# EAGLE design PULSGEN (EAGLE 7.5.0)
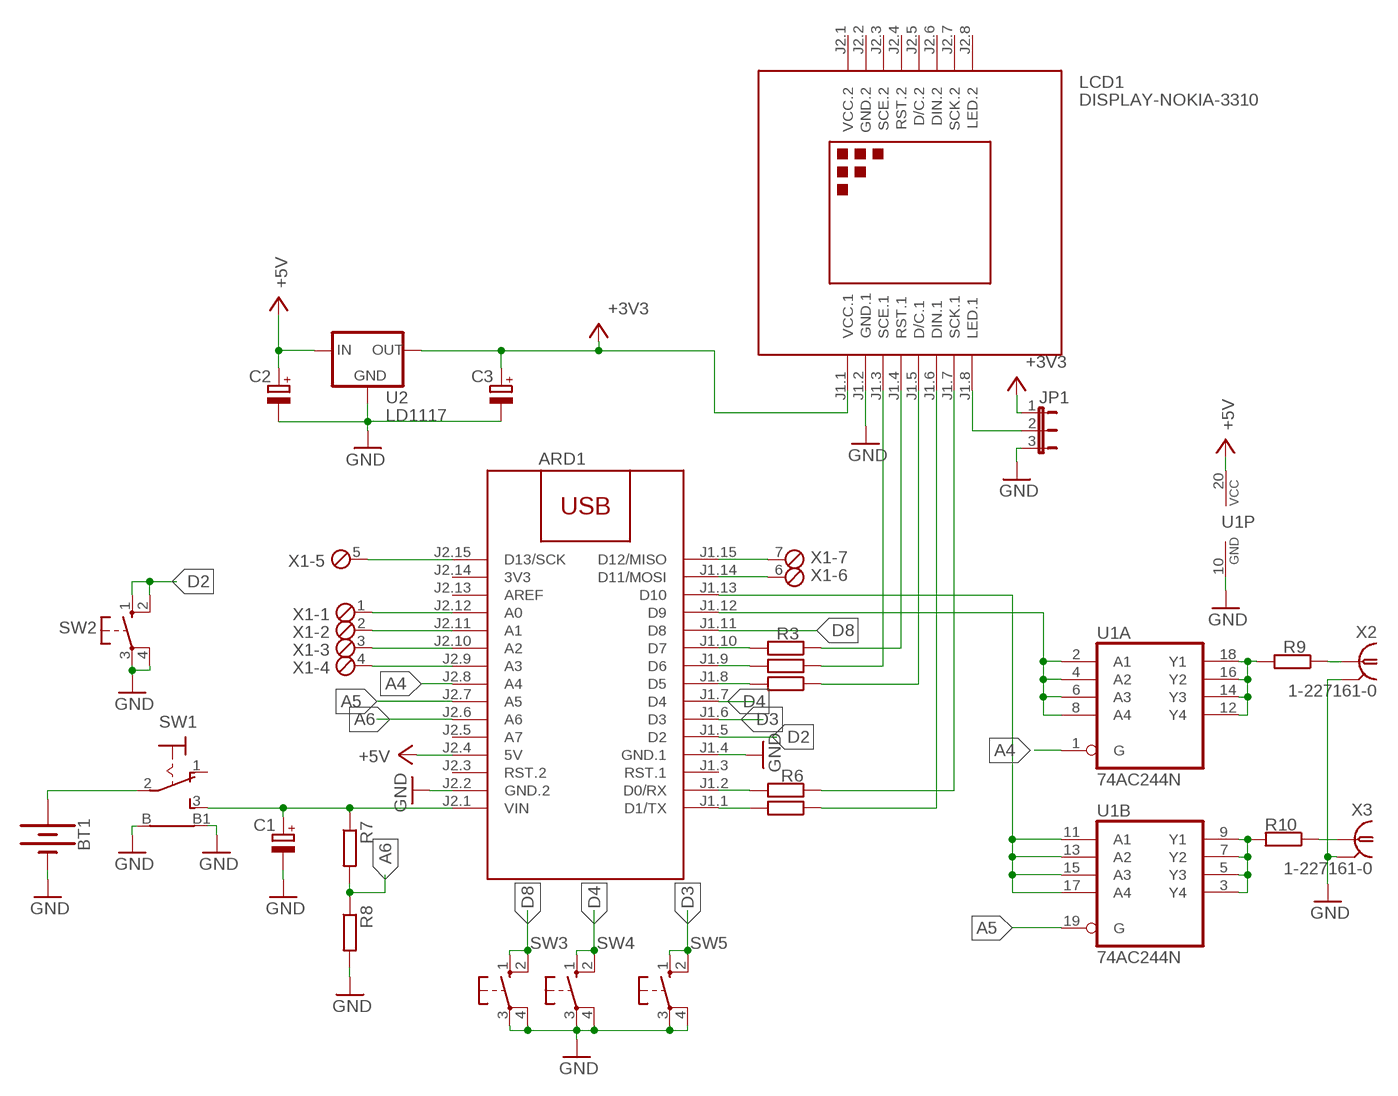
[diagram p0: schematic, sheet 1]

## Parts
ARD1  ARDUINO-NANO-3.0  [ARDUINO-NANO-3.0]
BT1  BATTERY-9V  [BATTCON_9V]
C1  CPOL-EUSMCC  [SMC_C]
C2  CPOL-EUSMCB  [SMC_B]
C3  CPOL-EUSMCB  [SMC_B]
JP1  JP2E  [JP2]
LCD1  DISPLAY-NOKIA-3310  [DISPLAY-NOKIA-3310]
R2  R-EU_R1206  [R1206]
R3  R-EU_R1206  [R1206]
R4  R-EU_R1206  [R1206]
R5  R-EU_R1206  [R1206]
R6  R-EU_R1206  [R1206]
R7  R-EU_R1206  [R1206]
R8  R-EU_R1206  [R1206]
R9  R-EU_R1206  [R1206]
R10  R-EU_R1206  [R1206]
SW1  9070-1W  [9070-1W]
SW2  40-XX  [B3F-40XX]
SW3  40-XX  [B3F-40XX]
SW4  40-XX  [B3F-40XX]
SW5  40-XX  [B3F-40XX]
U1  74AC244N  [DIL20]
U2  LD1117  [SOT223]
X1  MPT7  [7POL254]
X2  1-227161-0  [AMP_227161]
X3  1-227161-0  [AMP_227161]

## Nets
+3V3: C3.+ JP1.1 LCD1.J1.1(VCC.1) U2.2(OUT)
+5V: ARD1.J2.4(5V) C2.+ U1.20(P:VCC) U2.3(IN)
A4: ARD1.J2.8(A4) U1.1(A:G)
A5: ARD1.J2.7(A5) U1.19(B:G)
A6: ARD1.J2.6(A6) R7.2 R8.1
D2: ARD1.J1.5(D2) SW2.1(S) SW2.2(S1)
D3: ARD1.J1.6(D3) SW5.1(S) SW5.2(S1)
D4: ARD1.J1.7(D4) SW4.1(S) SW4.2(S1)
D8: ARD1.J1.11(D8) SW3.1(S) SW3.2(S1)
GND: ARD1.J1.4(GND.1) ARD1.J2.2(GND.2) BT1.- C1.- C2.- C3.- JP1.3 LCD1.J1.2(GND.1) R8.2 SW1.B SW1.B1 SW2.3(P) SW2.4(P1) SW3.3(P) SW3.4(P1) SW4.3(P) SW4.4(P1) SW5.3(P) SW5.4(P1) U1.10(P:GND) U2.1(GND) X2.2 X3.2
N$1: ARD1.J1.1(D1/TX) R5.2
N$2: LCD1.J1.6(DIN.1) R5.1
N$3: ARD1.J1.10(D7) R3.2
N$4: ARD1.J1.9(D6) R2.2
N$5: ARD1.J1.8(D5) R4.2
N$6: ARD1.J1.2(D0/RX) R6.2
N$7: ARD1.J2.12(A0) X1.1
N$8: LCD1.J1.4(RST.1) R3.1
N$9: LCD1.J1.3(SCE.1) R2.1
N$10: LCD1.J1.5(D/C.1) R4.1
N$11: ARD1.J2.11(A1) X1.2
N$12: LCD1.J1.7(SCK.1) R6.1
N$13: JP1.2 LCD1.J1.8(LED.1)
N$14: ARD1.J2.10(A2) X1.3
N$15: ARD1.J2.9(A3) X1.4
N$16: ARD1.J2.15(D13/SCK) X1.5
N$17: ARD1.J1.14(D11/MOSI) X1.6
N$18: ARD1.J1.15(D12/MISO) X1.7
N$19: R9.1 X2.1
N$20: ARD1.J1.12(D9) U1.2(A:A1) U1.4(A:A2) U1.6(A:A3) U1.8(A:A4)
N$21: ARD1.J1.13(D10) U1.11(B:A1) U1.13(B:A2) U1.15(B:A3) U1.17(B:A4)
N$22: R9.2 U1.12(A:Y4) U1.14(A:Y3) U1.16(A:Y2) U1.18(A:Y1)
N$23: R10.2 U1.3(B:Y4) U1.5(B:Y3) U1.7(B:Y2) U1.9(B:Y1)
N$24: BT1.+ SW1.2(P)
N$25: ARD1.J2.1(VIN) C1.+ R7.1 SW1.3(S)
N$26: R10.1 X3.1
Unconnected: ARD1.J1.3(RST.1) ARD1.J2.3(RST.2) ARD1.J2.5(A7) ARD1.J2.13(AREF) LCD1.J2.3(SCE.2) LCD1.J2.4(RST.2) LCD1.J2.5(D/C.2) LCD1.J2.6(DIN.2) LCD1.J2.7(SCK.2) LCD1.J2.8(LED.2) SW1.1(O)

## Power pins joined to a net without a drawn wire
3V3: ARD1.J2.14(3V3)
GND.2: LCD1.J2.2(GND.2)
VCC.2: LCD1.J2.1(VCC.2)

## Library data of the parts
ARD1 = diy-modules:ARDUINO-NANO-3.0: Arduino Nano 3.0 and compatible devices More details available here: https://www.arduino.cc/en/Main/ArduinoBoardNano Click here to find device on ebay.com
BT1 = SparkFun-Batteries:BATTERY: Battery - Single Cell; PROD_ID: BATT-10855
C1-C3 = rcl:CPOL-EU: POLARIZED CAPACITOR, European symbol
JP1 = jumper:JP2E: JUMPER
LCD1 = diy-modules:DISPLAY-NOKIA-3310: 84x48 Dot Matrix LCD Module based on Nokia 3310 display More details available here: https://arduinoandsoftware.wordpress.com/2012/12/30/nokia-33105110-3-3v-display-with-5v-arduino/
R2-R10 = rcl:R-EU_: RESISTOR, European symbol
SW1 = switch:9070-1W: TOGGLE SWITCH Marquardt
SW2-SW5 = switch-omron:40-XX: OMRON SWITCH; MF: OMRON COMPONENTS USA; MPN: B3F-4000; OC_FARNELL: 176434; OC_NEWARK: 36K3105
U1 = 74xx-eu:74*244: Octal BUFFER and LINE DRIVER, 3-state
U2 = v-reg:LD1117
X1 = con-phoenix-254:MPT7: PHOENIX CONNECTOR; OC_FARNELL: unknown; OC_NEWARK: unknown
X2 X3 = con-coax:?227161*: JACK, RIGHT ANGLE, 50 OHM, PCB, BNC; MF: TYCO ELECTRONICS; MPN: 1-227161; OC_FARNELL: unknown; OC_NEWARK: 33B3200

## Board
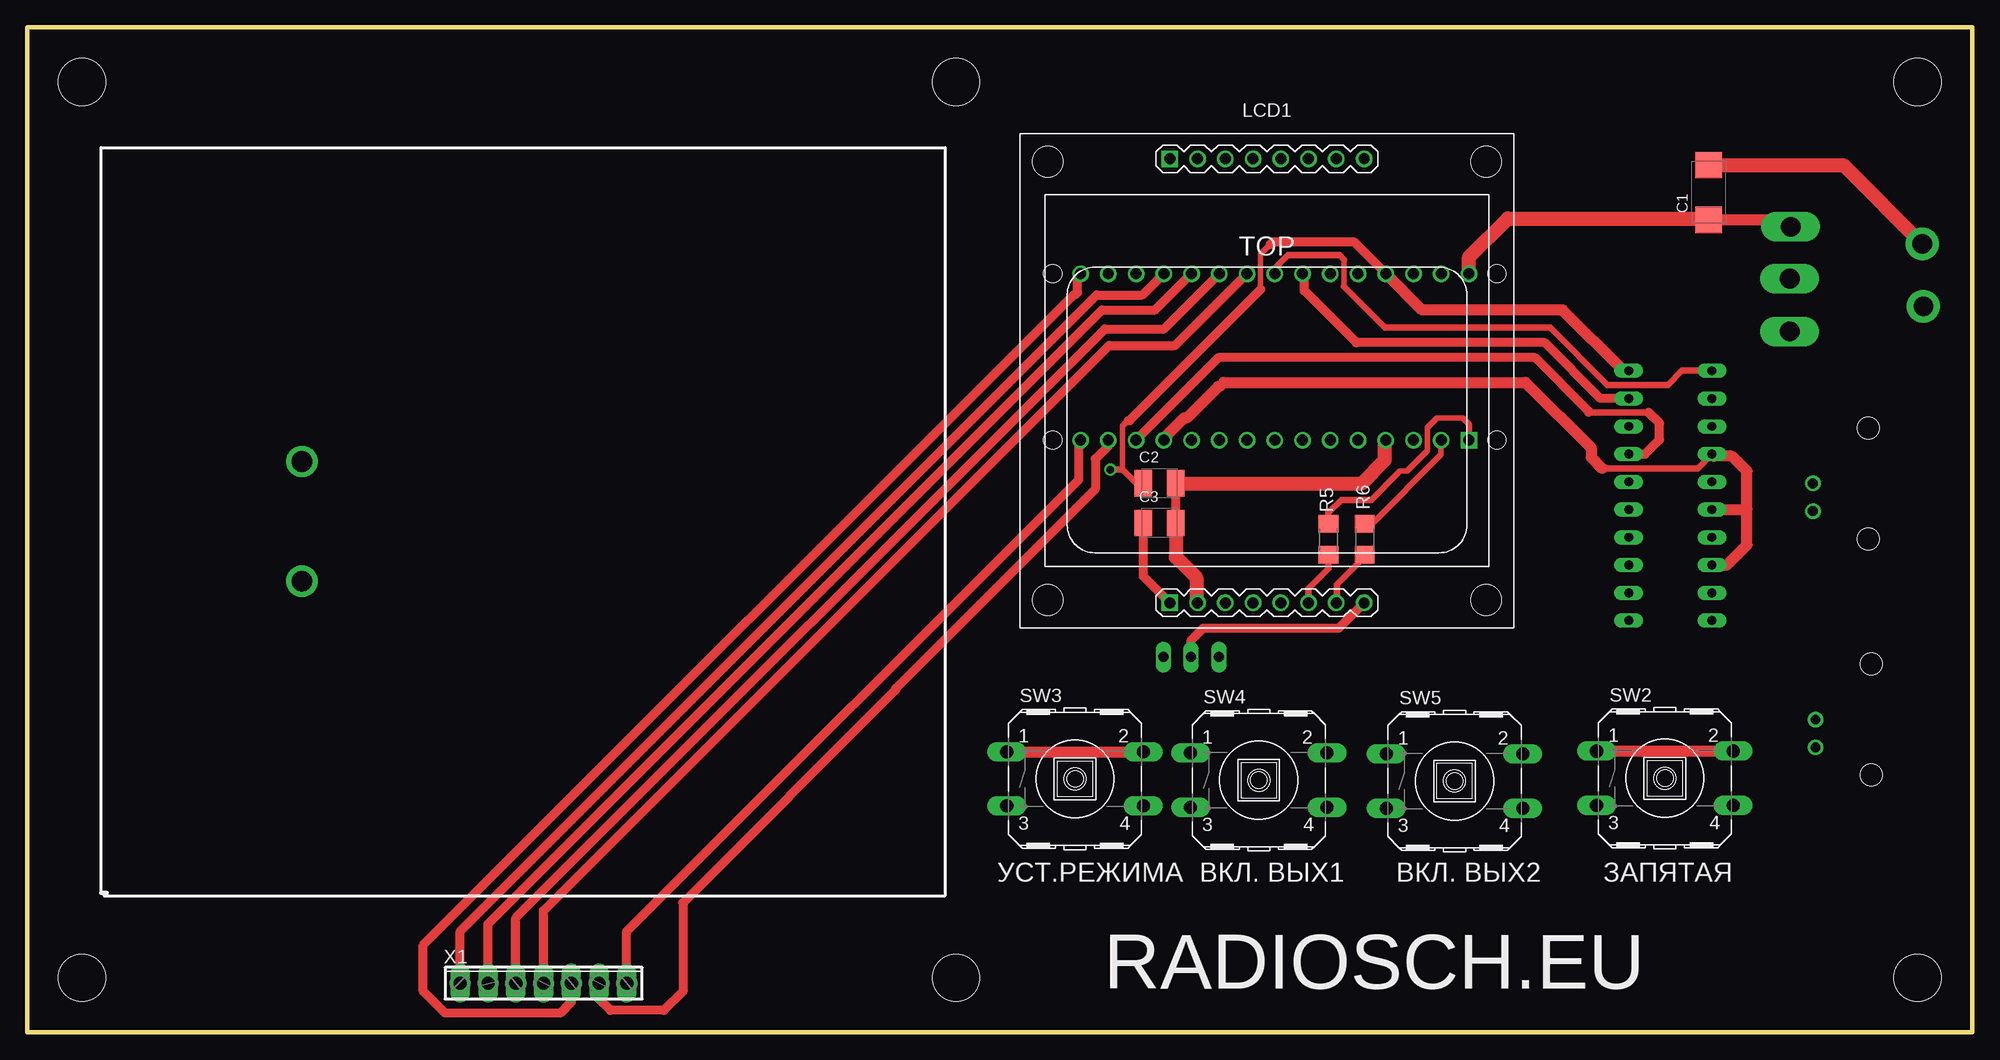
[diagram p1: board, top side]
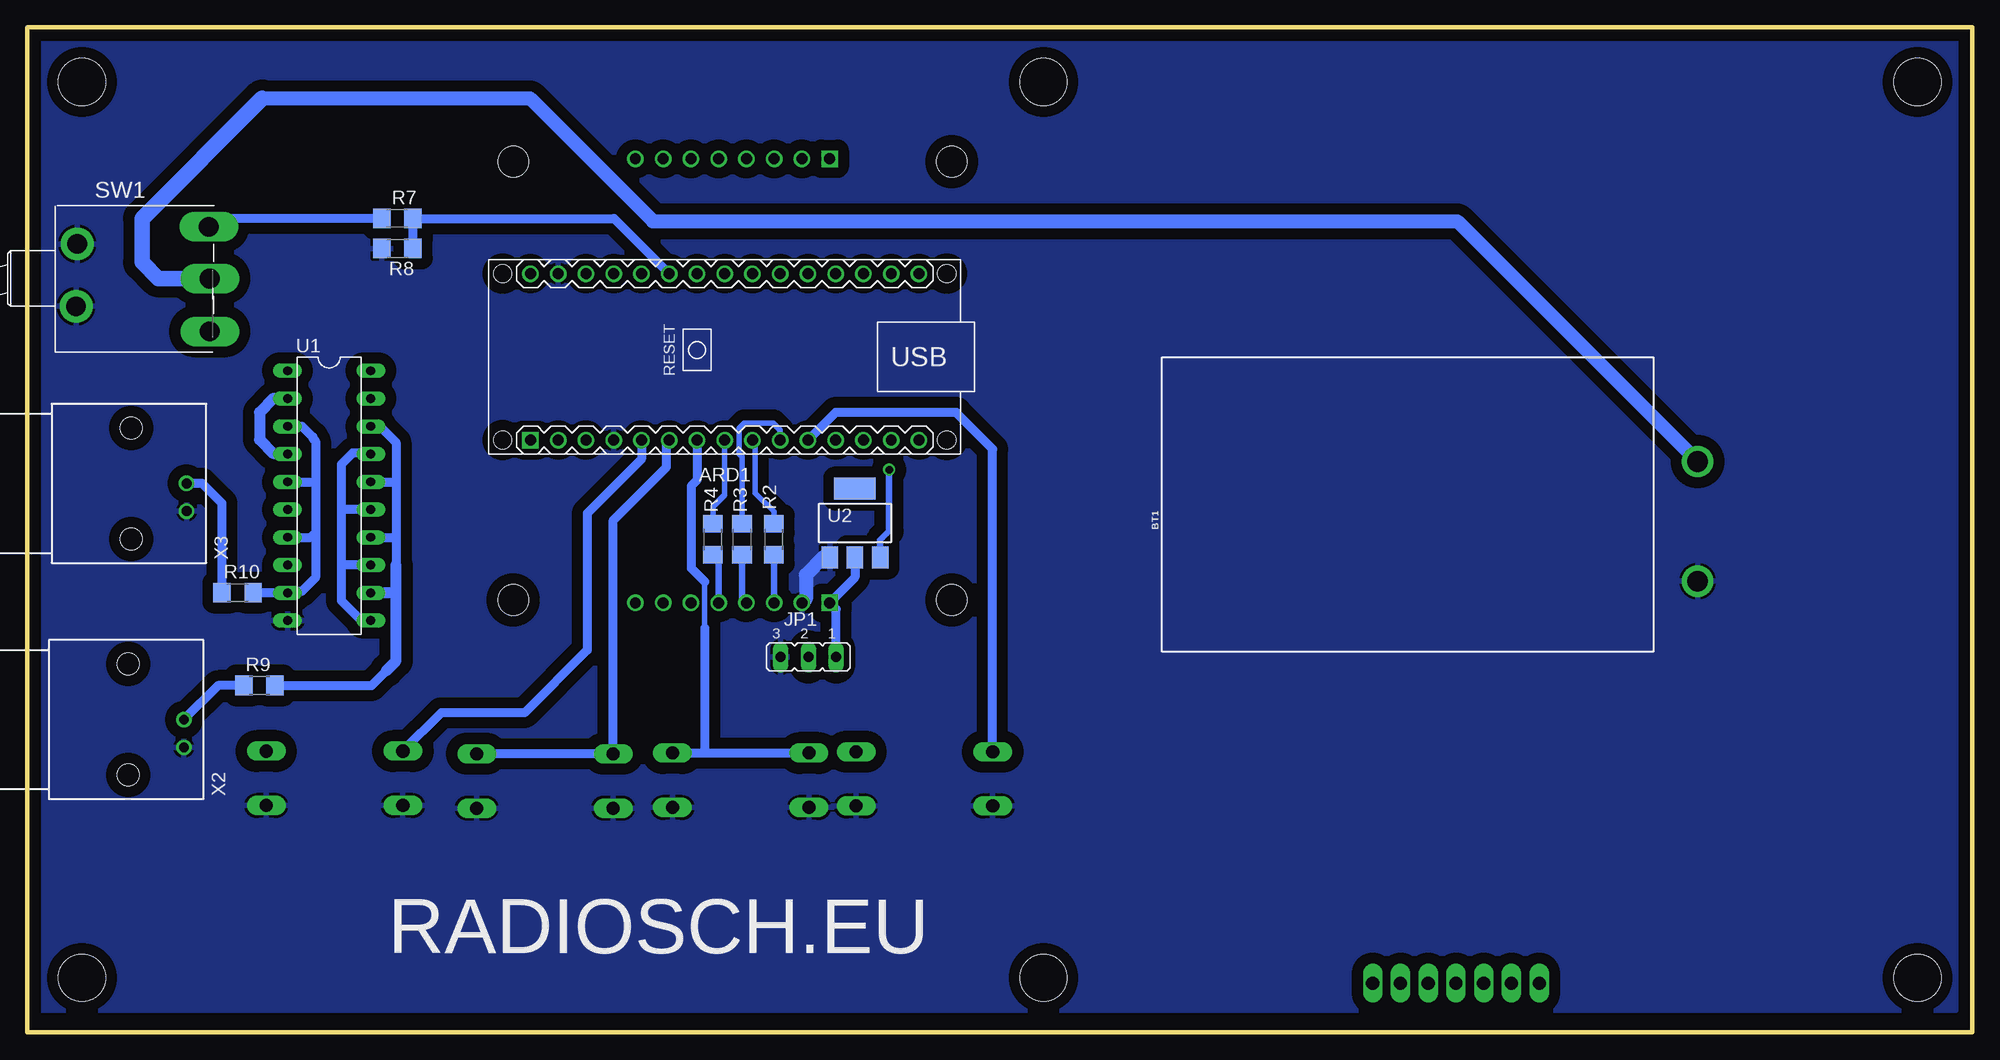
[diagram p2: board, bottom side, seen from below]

Size 178 x 92 mm. Coordinates in mm from the lower left corner, seen from the top.
Outline: 0,0 178,0 178,92 0,92 0,0
Copper layers (1*16): Top 0.035mm / dielectric 1.5mm / Bottom 0.035mm
Design rules "default": minimum track width 10mil, minimum drill 24mil, track to track 8mil, track to pad 8mil, pad to pad 8mil, via to via 8mil, smd to smd 8mil, copper to edge 40mil, drill to drill 8mil, minimum pad ring 10mil, minimum via ring 8mil, stop-mask expansion 4mil, vias tented up to drill 0mil, thermal gap 10mil
Holes 4.3 mm at 5,5 173,5 5,87 85,5 85,87 173,87

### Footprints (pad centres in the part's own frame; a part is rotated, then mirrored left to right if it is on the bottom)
ARDUINO-NANO-3.0 = drill 1 square: J1.1 17.78,7.62 | drill 1: J1.2 15.24,7.62; J1.3 12.7,7.62; J1.4 10.16,7.62; J1.5 7.62,7.62; J1.6 5.08,7.62; J1.7 2.54,7.62; J1.8 0,7.62; J1.9 -2.54,7.62; J1.10 -5.08,7.62; J1.11 -7.62,7.62; J1.12 -10.16,7.62; J1.13 -12.7,7.62; J1.14 -15.24,7.62; J1.15 -17.78,7.62; J2.1 17.78,-7.62; J2.2 15.24,-7.62; J2.3 12.7,-7.62; J2.4 10.16,-7.62; J2.5 7.62,-7.62; J2.6 5.08,-7.62; J2.7 2.54,-7.62; J2.8 0,-7.62; J2.9 -2.54,-7.62; J2.10 -5.08,-7.62; J2.11 -7.62,-7.62; J2.12 -10.16,-7.62; J2.13 -12.7,-7.62; J2.14 -15.24,-7.62; J2.15 -17.78,-7.62 | hole 1.651: -20.32,7.62; -20.32,-7.62; 20.32,-7.62; 20.32,7.62
BATTCON_9V = drill 1.905: + -4,-1; - -4,-11.954
SMC_C = smd 2.4 x 2.4: + -2.5,0; - 2.5,0
SMC_B = smd 1.6 x 2.4: + -1.5,0; - 1.5,0
JP2 = drill 0.914 long: 1 -2.54,0; 2 0,0; 3 2.54,0
DISPLAY-NOKIA-3310 = drill 1 square: J1.1 -8.89,-20.32; J2.1 -8.89,20.32 | drill 1: J1.2 -6.35,-20.32; J1.3 -3.81,-20.32; J1.4 -1.27,-20.32; J1.5 1.27,-20.32; J1.6 3.81,-20.32; J1.7 6.35,-20.32; J1.8 8.89,-20.32; J2.2 -6.35,20.32; J2.3 -3.81,20.32; J2.4 -1.27,20.32; J2.5 1.27,20.32; J2.6 3.81,20.32; J2.7 6.35,20.32; J2.8 8.89,20.32 | hole 2.8: -20.066,-20.066; 20.066,-20.066; 20.066,20.066; -20.066,20.066
R1206 = smd 1.6 x 1.803: 1 -1.422,0; 2 1.422,0
9070-1W = drill 1.813 long: 1 5.08,-4.835; 2 5.08,0 | drill 1.8 long: 3 4.98,4.735 | drill 1.8 pad 3: B -7.161,-2.544; B1 -7.061,3.167
B3F-40XX = drill 1.194 long: 1 -6.248,2.489; 2 6.248,2.489; 3 -6.248,-2.489; 4 6.248,-2.489
DIL20 = drill 0.813 long: 1 -11.43,-3.81; 2 -8.89,-3.81; 3 -6.35,-3.81; 4 -3.81,-3.81; 5 -1.27,-3.81; 6 1.27,-3.81; 7 3.81,-3.81; 8 6.35,-3.81; 9 8.89,-3.81; 10 11.43,-3.81; 11 11.43,3.81; 12 8.89,3.81; 13 6.35,3.81; 14 3.81,3.81; 15 1.27,3.81; 16 -1.27,3.81; 17 -3.81,3.81; 18 -6.35,3.81; 19 -8.89,3.81; 20 -11.43,3.81
SOT223 = smd 1.5 x 2: 1 -2.3,-3.15; 2 0,-3.15; 3 2.3,-3.15 | smd 3.8 x 2: 4 0,3.15
7POL254 = drill 1.2 long: 1 -7.62,0; 2 -5.08,0; 3 -2.54,0; 4 0,0; 5 2.54,0; 6 5.08,0; 7 7.62,0
AMP_227161 = drill 0.9 pad 1.27: 1 0,-5.08; 2 -2.54,-5.08 | hole 2: -5.08,0; 5.08,0

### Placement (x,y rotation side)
ARD1  114.17,61.83 180 bottom
BT1  21.12,53.25 0 bottom
C1  153.88,76.88 90 top
C2  103.62,50.25 0 top
C3  103.62,46.62 0 top
JP1  106.51,34.35 180 bottom
LCD1  113.46,59.64 0 top
R2  109.67,45.13 90 bottom
R3  112.59,45.13 90 bottom
R4  115.25,45.13 90 bottom
R5  119.08,45.13 90 top
R6  122.41,45.13 90 top
R7  144.12,74.5 0 bottom
R8  144.12,71.75 180 bottom
R9  156.75,31.75 0 bottom
R10  158.75,40.25 0 bottom
SW1  166.38,69 0 bottom
SW2  149.88,23.25 0 top
SW3  95.89,23.2 0 top
SW4  112.71,23.08 0 top
SW5  130.62,23 0 top
U1  150.38,49.12 270 bottom
U2  102.25,46.62 0 bottom
X1  47.25,4.5 0 top
X2  168.75,28.62 90 bottom
X3  168.5,50.25 90 bottom

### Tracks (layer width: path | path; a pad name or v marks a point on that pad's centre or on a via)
+3V3
  Top 0.813: C3.+ 102.12,41.77 LCD1.J1.1
  Bottom 0.813: JP1.1 103.97,38.72 LCD1.J1.1 102.25,41.64 U2.2
+5V  (via drill 0.7)
  Top 0.5: C2.+ 101.5,50.25 100.25,51.5 100.25,55.5 100.75,56 | 112.88,68 112.88,71.25 113.75,72.12
  Top 0.61: v99.12,51.5 100.25,51.5
  Top 0.813: 100.75,56 100.88,56 112.88,68 | 113.75,72.12 114,72.38 121.41,72.38 ARD1.J2.4
  Top 1.016: U1.20 146.07,60.55 140.5,66.12 127.66,66.12 ARD1.J2.4
  Bottom 0.61: U2.3 99.95,45.05 99.12,45.88 v99.12,51.5
A4
  Top 0.5: 120.5,68.25 120.5,70.75
  Top 0.61: U1.1 151.43,60.55 150.12,59.25 144.62,59.25 139.38,64.5 124.25,64.5 120.5,68.25 | ARD1.J2.8 114.25,69.53 114.25,70 115.38,71.12 120.12,71.12 120.5,70.75
A5
  Top 0.813: ARD1.J2.7 116.88,69.28 116.88,67.88 121.62,63.12 138.88,63.12 143.99,58.02 U1.19
A6
  Bottom 0.813: ARD1.J2.6 124.3,74.5 R7.2 R8.1
D2
  Top 1.016: SW2.1 SW2.2
  Bottom 0.813: ARD1.J1.5 121.79,52.46 126.75,47.5 126.75,35 132.5,29.25 140.12,29.25 SW2.1
D3
  Bottom 0.813: ARD1.J1.6 119.5,53.96 119.5,51.75 124.38,46.87 SW5.1 SW5.2
D4
  Bottom 0.5: 116,41.25 116,37
  Bottom 0.813: ARD1.J1.7 116.71,50.54 117.25,50 117.25,42.5 116,41.25 | 116,37 116,25.57 | SW4.2 116,25.57 | 116,25.57 SW4.1
D8
  Top 1.016: SW3.1 SW3.2
  Bottom 0.813: SW3.1 89.64,53.39 93,56.75 104.01,56.75 ARD1.J1.11
GND
  Top 0.813: C3.- C2.-
  Top 1.27: C2.- 122.12,50.25 124.25,52.38 124.25,54.13 ARD1.J1.4 | C3.- 105.12,43.5 107,41.62 107,39.43 LCD1.J1.2 | C1.- 166.23,79.38 SW1.B1
  Bottom 1.27: U2.1 105.15,43.48 106.75,41.88 106.75,39.68 LCD1.J1.2
  pour Bottom (isolate 1.016): 1.5,2 177,2 177,91 1.5,91
N$1
  Top 0.5: 125.5,51.25 125.62,51.38 126.25,51.38 128.12,53.25 128.12,55.38 129,56.25 131.38,56.25 132,55.62 132,54.26 ARD1.J1.1
  Top 0.61: R5.2 119.08,47.58 120.25,48.75 123,48.75 125.5,51.25
N$2
  Top 0.61: R5.1 119.08,42.45 117.25,40.62 117.25,39.34 LCD1.J1.6
N$3
  Bottom 0.5: R3.2 112.59,52.72 112.88,53 112.88,55.25 112.38,55.75 109.75,55.75 109.12,55.12 109.12,54.24 ARD1.J1.10
N$4
  Bottom 0.5: R2.2 109.67,47.67 111.38,49.38 111.38,53.95 ARD1.J1.9
N$5
  Bottom 0.5: ARD1.J1.8 114.17,49.2 115.25,48.12 R4.2
N$6
  Top 0.5: R6.2 123.05,46.55 129.38,52.88 129.38,54.17 ARD1.J1.2
N$7
  Top 0.813: X1.1 39.63,9.26 97.88,67.5 102.06,67.5 ARD1.J2.12
N$8
  Bottom 0.61: R3.1 112.59,39.72 LCD1.J1.4
N$9
  Bottom 0.61: R2.1 109.67,39.34 LCD1.J1.3
N$10
  Bottom 0.61: LCD1.J1.5 114.73,43.19 R4.1
N$11
  Top 0.813: X1.2 42.17,9.92 98.38,66.12 103.22,66.12 ARD1.J2.11
N$12
  Top 0.61: R6.1 122.41,43.53 119.88,41 119.88,39.38 LCD1.J1.7
N$13
  Top 0.813: JP1.2 106.51,35.88 107.62,37 120.03,37 LCD1.J1.8
N$14
  Top 0.813: X1.3 44.71,10.46 98.62,64.38 104.02,64.38 ARD1.J2.10
N$15
  Top 0.813: X1.4 47.25,11.12 99,62.88 105.06,62.88 ARD1.J2.9
N$16
  Top 0.813: X1.5 49.79,2.79 48.75,1.75 38.25,1.75 36.25,3.75 36.25,8 95.75,67.5 95.88,67.5 96.12,67.75 96.12,69.19 ARD1.J2.15
N$17
  Top 0.813: ARD1.J1.14 98.93,53.68 97.75,52.5 97.75,49.75 79.5,31.5 79.5,31.38 60,11.88 60,3.75 58.25,2 53.38,2 52.25,3.12 52.25,4.42 X1.6
N$18
  Top 0.813: X1.7 54.87,9.24 96.25,50.62 96.25,54.07 ARD1.J1.15
N$19
  Bottom 0.813: R9.1 160.54,31.75 X2.1
N$20
  Top 0.61: 144.12,51.62 152.88,51.62 U1.4
  Top 1.016: U1.8 155.53,42.77 157.38,44.62 157.38,47.88 | 157.38,47.88 157.38,51.38 156,52.75 154.37,52.75 U1.4 | U1.6 157.35,47.85 157.38,47.88 | ARD1.J1.12 104.01,54.38 105.88,56.25 106.12,56.25 109,59.12 109.12,59.12 109.5,59.5 137.12,59.5 143.12,53.5 143.12,52.62 144.12,51.62
  Bottom 1.016: U1.2 155.49,58.02 156.75,56.75 156.75,54.25 155.5,53 154.25,53 U1.4
N$21
  Top 0.61: 148.38,56.75 142.88,56.75
  Top 0.813: U1.17 148.06,52.94 149.38,54.25 149.38,55.75 148.38,56.75 | 142.88,56.75 142.88,56.88 138,61.75 109.01,61.75 ARD1.J1.13
  Bottom 0.813: U1.11 147.44,37.7 149.25,39.5 149.25,42.62 | 149.25,42.62 149.25,48 | 149.25,48 149.25,52 148.19,53.06 146.69,53.06 U1.17 | U1.15 149.1,47.85 149.25,48 | U1.13 149.1,42.77 149.25,42.62
N$22
  Bottom 0.813: U1.18 145.72,55.48 144.25,54 144.25,50.25 | 144.25,50.25 144.25,45.12 | 144.25,45.12 144.25,42.75 144.25,41.25 | 145.25,40.25 146.55,40.25 U1.12 | U1.16 144.4,50.4 144.25,50.25 | U1.14 144.44,45.31 144.25,45.12 | R9.2 146.5,31.75 145.12,33.12
  Bottom 1.016: 145.12,33.12 144.25,34 144.25,40.25 | 144.25,40.25 144.25,42.75 | 145.25,40.25 144.25,40.25
N$23
  Bottom 0.813: U1.3 152.85,55.48 151.88,54.5 151.88,54.38 151.62,54.12 151.62,50.62 | 151.62,50.62 151.62,45.75 | 151.62,45.75 151.62,41.62 152.88,40.38 154.04,40.38 U1.9 157.31,40.23 R10.2 | U1.7 152.06,45.31 151.62,45.75 | U1.5 151.85,50.4 151.62,50.62
N$24
  Bottom 1.27: 156.5,85.5 132,85.5 120.75,74.25 47.12,74.25 BT1.+
  Bottom 1.422: 156.5,85.5 167.5,74.5 167.5,70.5 166,69 SW1.2
N$25
  Top 1.016: C1.+ 160.75,74.38 SW1.3
  Top 1.27: ARD1.J2.1 131.95,70.95 135.5,74.5 153.75,74.5 C1.+
  Bottom 0.813: R7.1 160.63,74.5 SW1.3
N$26
  Bottom 0.813: R10.1 160.17,48.42 162,50.25 X3.1

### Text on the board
tPlace: УСТ.РЕЖИМА | ВКЛ. ВЫХ1 | ВКЛ. ВЫХ2 | ЗАПЯТАЯ | RADIOSCH.EU
bPlace: RADIOSCH.EU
